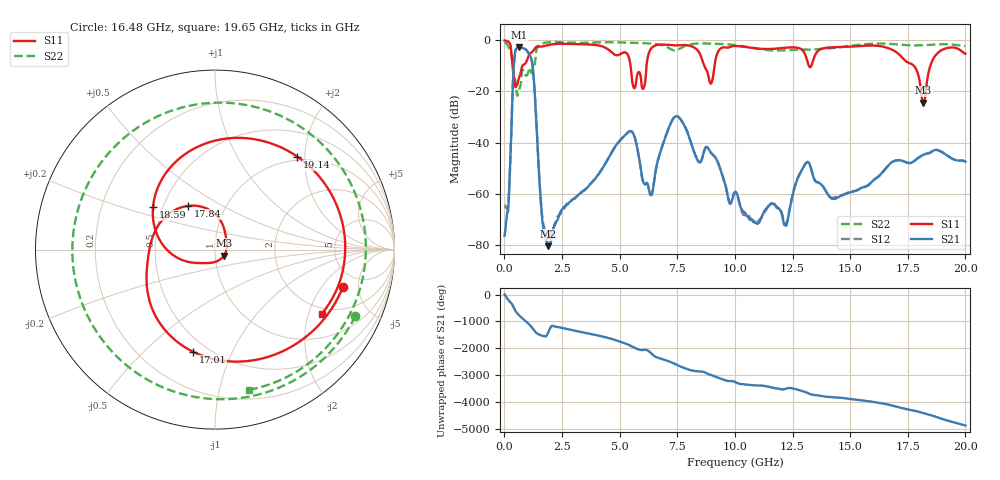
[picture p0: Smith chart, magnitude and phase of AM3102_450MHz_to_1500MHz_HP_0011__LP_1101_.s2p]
!Agilent Technologies,E8364B,MY43040894,A.07.50.67
!Agilent E8364B: A.07.50.67
!Date: Thursday, January 11, 2018 05:33:37
!Correction: S11(Full 2 Port(1,2))
!S21(Full 2 Port(1,2))
!S12(Full 2 Port(1,2))
!S22(Full 2 Port(1,2))
!S2P File: Measurements: S11, S21, S12, S22:
# Hz S  dB  R 50
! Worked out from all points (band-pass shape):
!   1601 points, 10 MHz to 20 GHz, reference 50 ohm
!   highest |S21| = -2.78 dB at 634.7 MHz (marker M1); lowest = -80.6 dB at 1.909 GHz (marker M2)
!   |S21| within 3 dB of the highest: 447.2 MHz to 1.097 GHz (649.8 MHz wide, 84.2 % of centre)
!   lowest |S11| = -24.4 dB at 18.18 GHz (marker M3), VSWR 1.13, Z = 55.2 - j3.65 ohm
!   |S11| at or under -10 dB: 5.474 GHz to 6.166 GHz (692 MHz wide, 11.9 % of centre); 8.674 GHz to 9.113 GHz (438.8 MHz wide, 4.93 % of centre); 17.77 GHz to 18.48 GHz (710.1 MHz wide, 3.92 % of centre)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
!   |S22| runs from -21.7 to -0.7 dB; largest |S21 - S12| = 0.0027
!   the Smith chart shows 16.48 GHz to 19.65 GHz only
!   S11 on the Smith chart (normalised r, x): 16.48 GHz: 3.56, -3.31; 17.01 GHz: 0.42, -0.72; 17.84 GHz: 0.67, +0.35; 18.59 GHz: 0.44, +0.26; 19.14 GHz: 0.93, +1.85; 19.65 GHz: 1.77, -2.44
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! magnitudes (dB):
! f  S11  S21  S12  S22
! 10 MHz  0.0  -76.5  -64.6  -0.7
! 184.9 MHz  -0.6  -62.9  -62.2  -2.7
! 434.8 MHz  -16.1  -6.8  -6.8  -14.0
! 634.7 MHz  -14.8  -2.8  -2.8  -19.5
! 1.197 GHz  -4.6  -8.4  -8.4  -12.7
! 1.909 GHz  -1.8  -80.6  -78.1  -0.8
! 3.346 GHz  -1.5  -59.5  -59.4  -1.0
! 6.019 GHz  -19.0  -55.3  -55.2  -1.1
! 6.682 GHz  -1.8  -46.2  -46.2  -1.6
! 7.519 GHz  -2.0  -29.8  -29.8  -3.7
! 10.01 GHz  -2.2  -59.3  -59.4  -1.9
! 12.19 GHz  -2.9  -72.4  -72.0  -3.9
! 13.34 GHz  -9.5  -51.4  -51.3  -3.7
! 16.48 GHz  -2.6  -50.8  -50.9  -1.3
! 16.68 GHz  -3.1  -48.7  -48.7  -1.3
! 17.01 GHz  -4.7  -46.9  -47.0  -1.6
! 17.84 GHz  -10.9  -46.8  -46.8  -2.0
! 18.18 GHz  -24.4  -44.8  -44.9  -1.9
! 18.59 GHz  -7.5  -43.3  -43.2  -1.7
! 19.14 GHz  -3.2  -44.6  -44.6  -1.5
! 19.65 GHz  -3.2  -47.0  -47.0  -1.9
! 20 GHz  -5.2  -47.5  -47.3  -2.3
